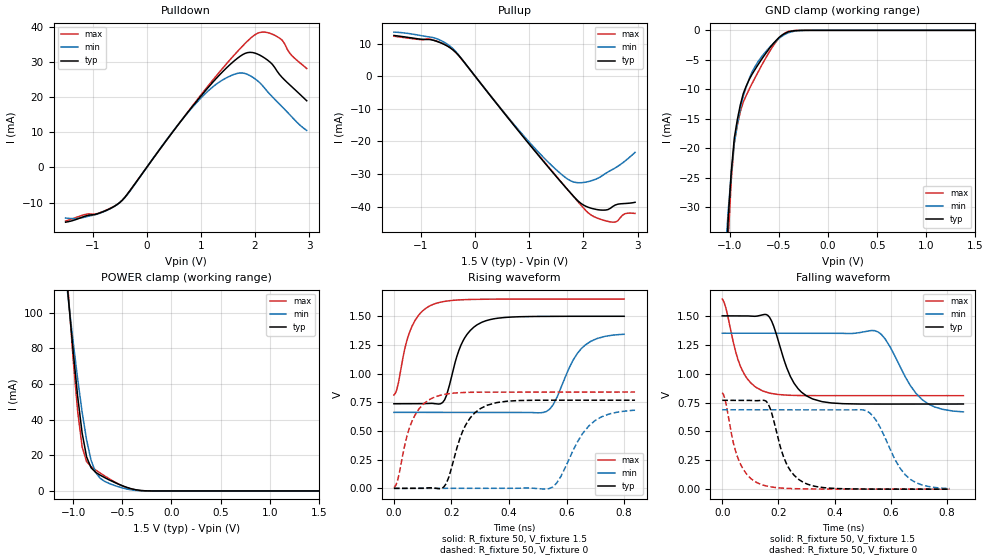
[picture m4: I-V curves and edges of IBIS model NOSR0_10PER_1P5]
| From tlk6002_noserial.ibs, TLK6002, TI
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[Model]   NOSR0_10PER_1P5
Model_type   3-state
Polarity   Non-Inverting
Enable   Active-Low
Cref =  15.0000pF
Rref =  100.0000M
Vref =  0V
Vmeas =  0.75
C_comp   2.108887p   1.924381p   2.428843p
[Temperature Range]   25   125   -40
[Voltage Range]   1.5   1.35   1.65
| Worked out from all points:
|   slope of the pulldown table from 0 to 0.225 V, typ, clamps not added: 47.1 ohm
|   slope of the pullup table from 0 to 0.225 V, typ, clamps not added: 47 ohm
|   GND clamp passes 1 mA (typ) near -0.48 V on its own axis
|   POWER clamp passes 1 mA (typ) near -0.39 V on its own axis
|   rising waveform, R_fixture 50, V_fixture 1.5: 20-80 % time 63.7ps typ, 79.7ps min, 57.8ps max; typ from 0.737 V to 1.5 V
|   rising waveform, R_fixture 50, V_fixture 0: 20-80 % time 67.8ps typ, 90.9ps min, 59.8ps max; typ from 0 V to 0.769 V
|   falling waveform, R_fixture 50, V_fixture 1.5: 20-80 % time 71.9ps typ, 97.8ps min, 61.7ps max; typ from 1.5 V to 0.738 V
|   falling waveform, R_fixture 50, V_fixture 0: 20-80 % time 63.6ps typ, 86.9ps min, 57.1ps max; typ from 0.769 V to 0.001 V
[POWER_clamp]
-1.5V     423.5mA    352.2mA    503mA
-1.061V   115.6mA    113mA      119.8mA
-1.045V   105.8mA    105.4mA    107.7mA
-1V       78.14mA    83.49mA    73.84mA
-954.5mV  53.09mA    62.89mA    44.72mA
-909.1mV  32.54mA    44.27mA    24.77mA
-863.6mV  19.13mA    28.63mA    16.48mA
-818.2mV  13.01mA    17.22mA    13.64mA
-772.7mV  10.47mA    10.51mA    11.79mA
-681.8mV  7.535mA    5.431mA    8.488mA
-318.2mV  297uA      112.4uA    206.1uA
1.5V      31.47nA    84.52nA    126.1nA
[Pulldown]
-1.5V     -15.59mA   -14.4mA    -15.27mA
-909.1mV  -13.19mA   -13.27mA   -13.12mA
-454.5mV  -9.369mA   -9.419mA   -9.379mA
909.1mV   18.53mA    18.18mA    18.76mA
1.273V    25.07mA    23.48mA    25.76mA
1.636V    30.51mA    26.53mA    32.26mA
1.909V    32.66mA    26.03mA    36.57mA
2.045V    32.18mA    24.59mA    38.07mA
2.227V    30.5mA     21.57mA    38.29mA
2.5V      25.54mA    17.21mA    36.13mA
2.682V    22.85mA    14.28mA    31.72mA
2.955V    18.91mA    10.48mA    28.08mA
[Pullup]
-1.5V     12.5mA     13.54mA    12.26mA
-772.7mV  11.03mA    11.84mA    11.09mA
-409.1mV  8.07mA     8.448mA    8.113mA
-227.3mV  4.842mA    4.891mA    4.759mA
1V        -20.87mA   -20.22mA   -20.66mA
1.455V    -29.92mA   -28.02mA   -29.78mA
1.773V    -36mA      -32.16mA   -36.04mA
2.045V    -39.91mA   -32.5mA    -41.22mA
2.364V    -41.09mA   -30.34mA   -44.15mA
2.591V    -39.51mA   -28.12mA   -44.74mA
2.773V    -39.06mA   -25.98mA   -42.17mA
2.955V    -38.69mA   -23.37mA   -42.1mA
[GND_clamp]
-1.5V     -337mA     -245.7mA   -453.6mA
-1.045V   -41.26mA   -37.73mA   -47.59mA
-1.015V   -31.48mA   -30.32mA   -34.73mA
-984.8mV  -23.81mA   -24.11mA   -25.24mA
-954.5mV  -18.25mA   -19.11mA   -19.1mA
-893.9mV  -12.68mA   -13.3mA    -13.81mA
-863.6mV  -10.74mA   -11.17mA   -12.17mA
-772.7mV  -7.41mA    -7.007mA   -8.984mA
-712.1mV  -5.806mA   -5.299mA   -7.049mA
-560.6mV  -2.304mA   -2.277mA   -2.676mA
-439.4mV  -510.4uA   -690.3uA   -461.4uA
1.5V      31.47nA    1.543uA    64.91nA
[Ramp]
dV/dt_f  0.3875845/57.03604p   0.3555494/81.06509p   0.4227658/48.54158p
dV/dt_r  0.3862979/53.35571p   0.347329/74.52028p   0.4206851/46.83571p
R_load = 50
[Rising Waveform]
R_fixture = 50
V_fixture = 1.5
V_fixture_min = 1.35
V_fixture_max = 1.65
0s        737.4mV    662.6mV    813.7mV
10ps      737.4mV    662.6mV    860.8mV
62ps      737.3mV    662.6mV    1.408V
133ps     740.9mV    662.6mV    1.6V
176ps     771.1mV    662.6mV    1.63V
238ps     1.276V     662.6mV    1.644V
306ps     1.448V     662.6mV    1.649V
531ps     1.499V     671.9mV    1.65V
650ps     1.5V       1.215V     1.65V
800ps     1.5V       1.343V     1.65V
[Rising Waveform]
R_fixture = 50
V_fixture = 0
V_fixture_min = 0
V_fixture_max = 0
0s        3.061uV    1.074uV    6.418mV
14ps      4.648uV    1.072uV    81.23mV
64ps      -60.38uV   1.067uV    592.5mV
142ps     1.813mV    1.059uV    797.3mV
182ps     42.71mV    1.054uV    822.2mV
255ps     576.8mV    -1.192uV   837mV
324ps     724.8mV    38.26uV    838.8mV
552ps     768.6mV    12.22mV    839.1mV
676ps     768.4mV    541.2mV    839.4mV
838ps     768.5mV    680.8mV    839.7mV
[Falling Waveform]
R_fixture = 50
V_fixture = 1.5
V_fixture_min = 1.35
V_fixture_max = 1.65
0s        1.5V       1.35V      1.645V
68ps      1.5V       1.35V      1.045V
100ps     1.498V     1.35V      923.7mV
144ps     1.51V      1.35V      850mV
176ps     1.454V     1.35V      828.3mV
254ps     924.7mV    1.35V      811.9mV
321ps     782.2mV    1.35V      810mV
554ps     737.1mV    1.363V     809.9mV
710ps     737.5mV    779.6mV    809.9mV
859ps     737.6mV    669.6mV    809.8mV
[Falling Waveform]
R_fixture = 50
V_fixture = 0
V_fixture_min = 0
V_fixture_max = 0
0s        769.5mV    687.7mV    835.2mV
56ps      769.5mV    687.7mV    267.7mV
132ps     767.9mV    687.7mV    48.23mV
163ps     741.1mV    687.7mV    25.59mV
226ps     234.8mV    687.7mV    8.229mV
288ps     60.78mV    687.7mV    3.777mV
514ps     1.983mV    678.4mV    1.708mV
550ps     1.676mV    589mV      1.649mV
651ps     1.288mV    127.2mV    1.46mV
810ps     1.135mV    6.849mV    1.15mV
